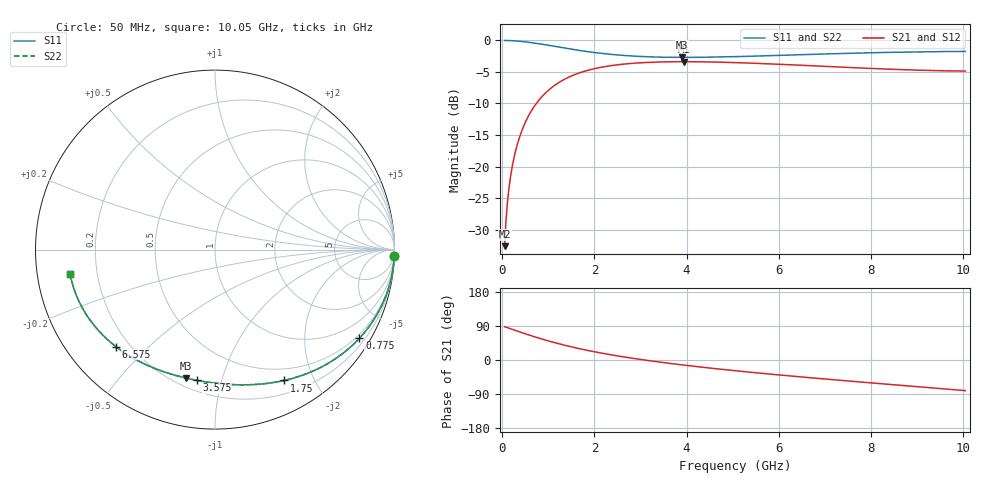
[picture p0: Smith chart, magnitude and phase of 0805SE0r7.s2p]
! AVX Thin Film Operation		Date: August 2001
! Description: Accu-P® Series, Thin Film, SMD, RF Capacitor
! Part Number: 08051J0R7ABT
! 50 MHz  -  10.05 GHz
! Serial Measurements
# mhz S db R 50
!	S11		S21		S12		S22
!	dB	Phase	dB	Phase	dB	Phase	dB	Phase
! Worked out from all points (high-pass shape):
!   401 points, 50 MHz to 10.05 GHz, reference 50 ohm
!   highest |S21| = -3.37 dB at 3.95 GHz (marker M1); lowest = -32.6 dB at 50 MHz (marker M2)
!   |S21| within 3 dB of the highest: 1.297 GHz to end of sweep
!   lowest |S11| = -2.7 dB at 3.9 GHz (marker M3), VSWR 6.52, Z = 12.4 - j38.4 ohm
!   |S11| at or under -10 dB: nowhere
!   |S22| runs from -2.7 to 0.0 dB; largest |S21 - S12| = 0
!   S11 on the Smith chart (normalised r, x): 50 MHz: 0, -54; 775 MHz: 0.38, -3.50; 1.75 GHz: 0.35, -1.61; 3.575 GHz: 0.26, -0.83; 6.575 GHz: 0.15, -0.40; 10.05 GHz: 0.10, -0.08
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50  -0.00 -2.1  -32.63 87.9  -32.63 87.9  -0.00 -2.1
75  -0.01 -3.2  -29.12 86.8  -29.12 86.8  -0.01 -3.2
125  -0.01 -5.3  -24.69 84.7  -24.69 84.7  -0.01 -5.3
175  -0.03 -7.5  -21.79 82.5  -21.79 82.5  -0.03 -7.5
225  -0.05 -9.6  -19.64 80.4  -19.64 80.4  -0.05 -9.6
300  -0.08 -12.7  -17.20 77.3  -17.20 77.3  -0.08 -12.7
400  -0.15 -16.9  -14.80 73.1  -14.80 73.1  -0.15 -16.9
500  -0.22 -20.9  -12.99 69.1  -12.99 69.1  -0.22 -20.9
775  -0.50 -31.6  -9.64 58.4  -9.64 58.4  -0.50 -31.6
1200  -1.02 -46.3  -6.80 43.7  -6.80 43.7  -1.02 -46.3
1725  -1.64 -61.4  -5.02 28.6  -5.02 28.6  -1.64 -61.4
1750  -1.67 -62.1  -4.96 27.9  -4.96 27.9  -1.67 -62.1
2500  -2.30 -79.2  -3.86 10.8  -3.86 10.8  -2.30 -79.2
3400  -2.64 -95.2  -3.42 -5.3  -3.42 -5.3  -2.64 -95.2
3575  -2.67 -98.0  -3.39 -8.0  -3.39 -8.0  -2.67 -98.0
3900  -2.69 -102.8  -3.37 -12.9  -3.37 -12.9  -2.69 -102.8
3950  -2.69 -103.6  -3.37 -13.6  -3.37 -13.6  -2.69 -103.6
5050  -2.57 -118.2  -3.51 -28.2  -3.51 -28.2  -2.57 -118.2
6575  -2.24 -135.6  -3.96 -45.6  -3.96 -45.6  -2.24 -135.6
6725  -2.21 -137.2  -4.02 -47.2  -4.02 -47.2  -2.21 -137.2
8400  -1.89 -154.2  -4.56 -64.4  -4.56 -64.4  -1.89 -154.2
10050  -1.74 -170.6  -4.86 -80.8  -4.86 -80.8  -1.74 -170.6
